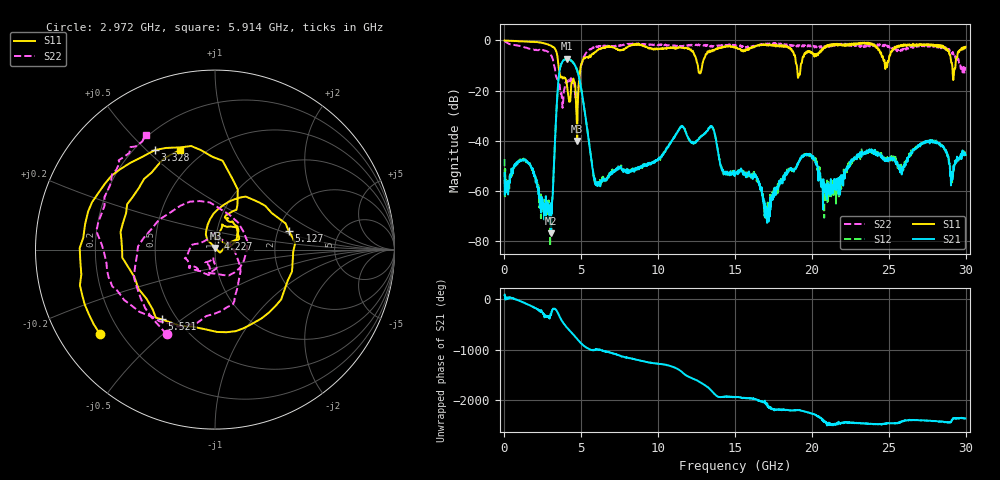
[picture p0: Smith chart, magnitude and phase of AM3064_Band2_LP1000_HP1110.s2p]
# Hz S DB R 50.0
!freq dBS11 angS11 dBS21 angS21 dBS12 angS12 dBS22 angS22
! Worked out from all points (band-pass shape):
!   1600 points, 10 MHz to 29.98 GHz, reference 50 ohm
!   highest |S21| = -7.32 dB at 4.077 GHz (marker M1); lowest = -76.7 dB at 3.028 GHz (marker M2)
!   |S21| within 3 dB of the highest: 3.645 GHz to 4.625 GHz (980.6 MHz wide, 23.7 % of centre)
!   lowest |S11| = -40.0 dB at 4.733 GHz (marker M3), VSWR 1.02, Z = 50.2 + j0.973 ohm
!   |S11| at or under -10 dB: 3.514 GHz to 4.971 GHz (1.456 GHz wide, 34.3 % of centre); 12.58 GHz to 12.86 GHz (283.3 MHz wide, 2.23 % of centre); 19.01 GHz to 19.27 GHz (259.2 MHz wide, 1.35 % of centre)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
!   |S22| runs from -26.8 to -0.3 dB; largest |S21 - S12| = 0.012
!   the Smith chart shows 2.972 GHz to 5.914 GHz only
!   S11 on the Smith chart (normalised r, x): 2.972 GHz: 0.13, -0.32; 3.328 GHz: 0.28, +0.53; 4.227 GHz: 1.03, +0.12; 5.127 GHz: 2.28, +0.59; 5.521 GHz: 0.41, -0.42; 5.914 GHz: 0.38, +0.64
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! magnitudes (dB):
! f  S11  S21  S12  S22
! 10 MHz  0.0  -52.7  -47.2  -0.3
! 1.472 GHz  -0.5  -48.5  -48.1  -3.1
! 2.972 GHz  -2.0  -73.1  -81.9  -5.3
! 3.028 GHz  -2.1  -76.7  -66.2  -5.9
! 3.328 GHz  -3.8  -34.6  -34.5  -13.6
! 3.609 GHz  -13.7  -11.3  -11.2  -18.8
! 4.077 GHz  -18.4  -7.3  -7.4  -16.6
! 4.227 GHz  -24.1  -7.6  -7.6  -16.8
! 4.733 GHz  -40.0  -12.0  -11.9  -23.1
! 5.015 GHz  -9.2  -20.1  -20.1  -9.7
! 5.127 GHz  -7.5  -24.6  -24.6  -7.1
! 5.521 GHz  -6.2  -41.5  -41.4  -3.8
! 5.914 GHz  -4.6  -57.3  -55.9  -2.5
! 10 GHz  -3.4  -47.1  -47.0  -1.8
! 13.43 GHz  -4.4  -34.1  -34.2  -2.3
! 15 GHz  -2.7  -53.0  -53.1  -1.9
! 16.39 GHz  -2.1  -54.2  -54.7  -2.2
! 17.07 GHz  -2.1  -71.3  -68.0  -1.5
! 19.99 GHz  -4.8  -46.0  -46.0  -2.0
! 20.91 GHz  -2.3  -61.0  -61.7  -2.4
! 25 GHz  -8.0  -46.9  -46.9  -2.2
! 29.98 GHz  -2.6  -45.6  -45.8  -10.6
